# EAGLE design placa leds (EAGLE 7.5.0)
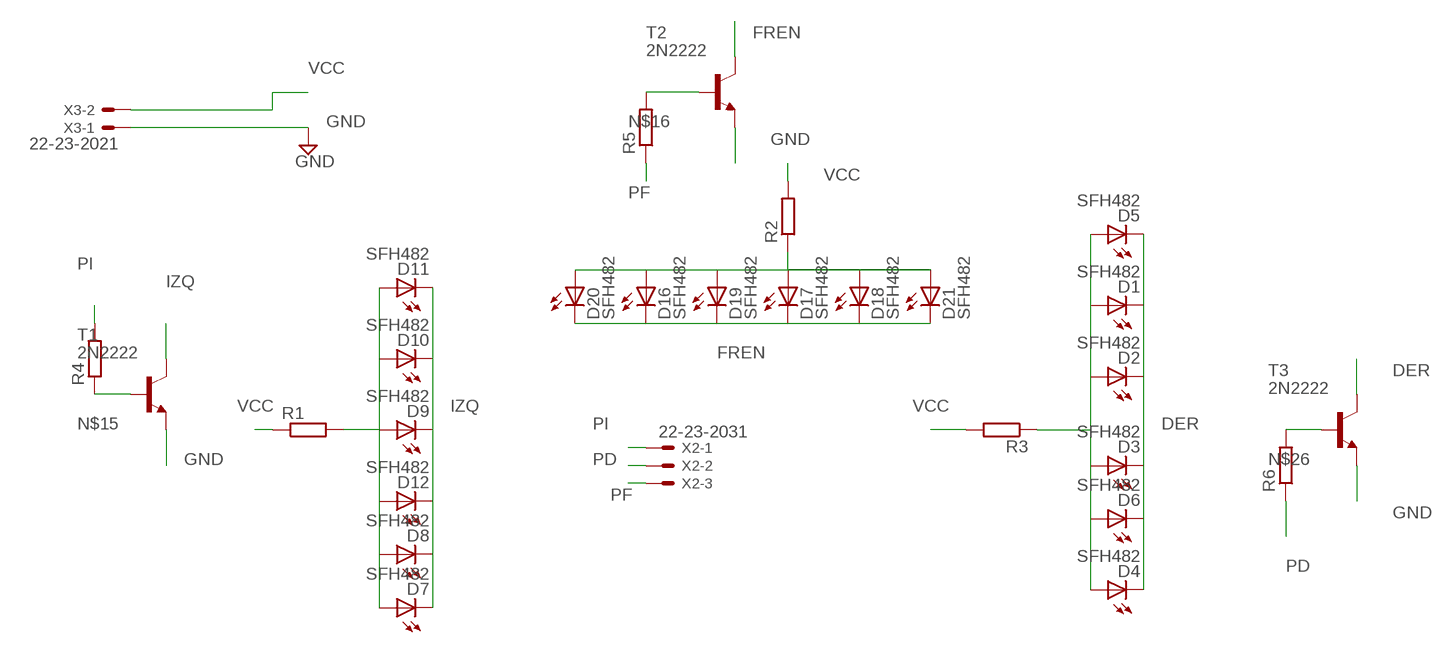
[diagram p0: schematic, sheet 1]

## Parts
D1  SFH482  [SFH482]
D2  SFH482  [SFH482]
D3  SFH482  [SFH482]
D4  SFH482  [SFH482]
D5  SFH482  [SFH482]
D6  SFH482  [SFH482]
D7  SFH482  [SFH482]
D8  SFH482  [SFH482]
D9  SFH482  [SFH482]
D10  SFH482  [SFH482]
D11  SFH482  [SFH482]
D12  SFH482  [SFH482]
D16  SFH482  [SFH482]
D17  SFH482  [SFH482]
D18  SFH482  [SFH482]
D19  SFH482  [SFH482]
D20  SFH482  [SFH482]
D21  SFH482  [SFH482]
R1  R-EU_VTA54  [VTA54]
R2  R-EU_VTA54  [VTA54]
R3  R-EU_VTA54  [VTA54]
R4  R-EU_0204/7  [0204/7]
R5  R-EU_0204/7  [0204/7]
R6  R-EU_0204/7  [0204/7]
T1  2N2222  [TO18]
T2  2N2222  [TO18]
T3  2N2222  [TO18]
X2  22-23-2031  [22-23-2031]
X3  22-23-2021  [22-23-2021]

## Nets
DER: D1.K(C) D2.K(C) D3.K(C) D4.K(C) D5.K(C) D6.K(C) T3.3(C)
FREN: D16.K(C) D17.K(C) D18.K(C) D19.K(C) D20.K(C) D21.K(C) T2.3(C)
GND: T1.1(E) T2.1(E) T3.1(E) X3.1
IZQ: D7.K(C) D8.K(C) D9.K(C) D10.K(C) D11.K(C) D12.K(C) T1.3(C)
N$2: D7.A D8.A D9.A D10.A D11.A D12.A R1.2
N$3: D16.A D17.A D18.A D19.A D20.A D21.A R2.1
N$4: D1.A D2.A D3.A D4.A D5.A D6.A R3.1
N$15: R4.1 T1.2(B)
N$16: R5.2 T2.2(B)
N$26: R6.2 T3.2(B)
PD: R6.1 X2.2
PF: R5.1 X2.3
PI: R4.2 X2.1
VCC: R1.1 R2.2 R3.2 X3.2

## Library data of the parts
D1-D12 D16-D21 = led:SFH482: IR LED
R1-R6 = resistor:R-EU_: RESISTOR, European symbol
T1-T3 = transistor:2N2222: NPN TRANSISTOR
X2 = con-molex:22-23-2031: .100" (2.54mm) Center Header - 3 Pin; MF: MOLEX; MPN: 22-23-2031; OC_FARNELL: 1462950; OC_NEWARK: 30C0862
X3 = con-molex:22-23-2021: .100" (2.54mm) Center Header - 2 Pin; MF: MOLEX; MPN: 22-23-2021; OC_FARNELL: 1462926; OC_NEWARK: 25C3832

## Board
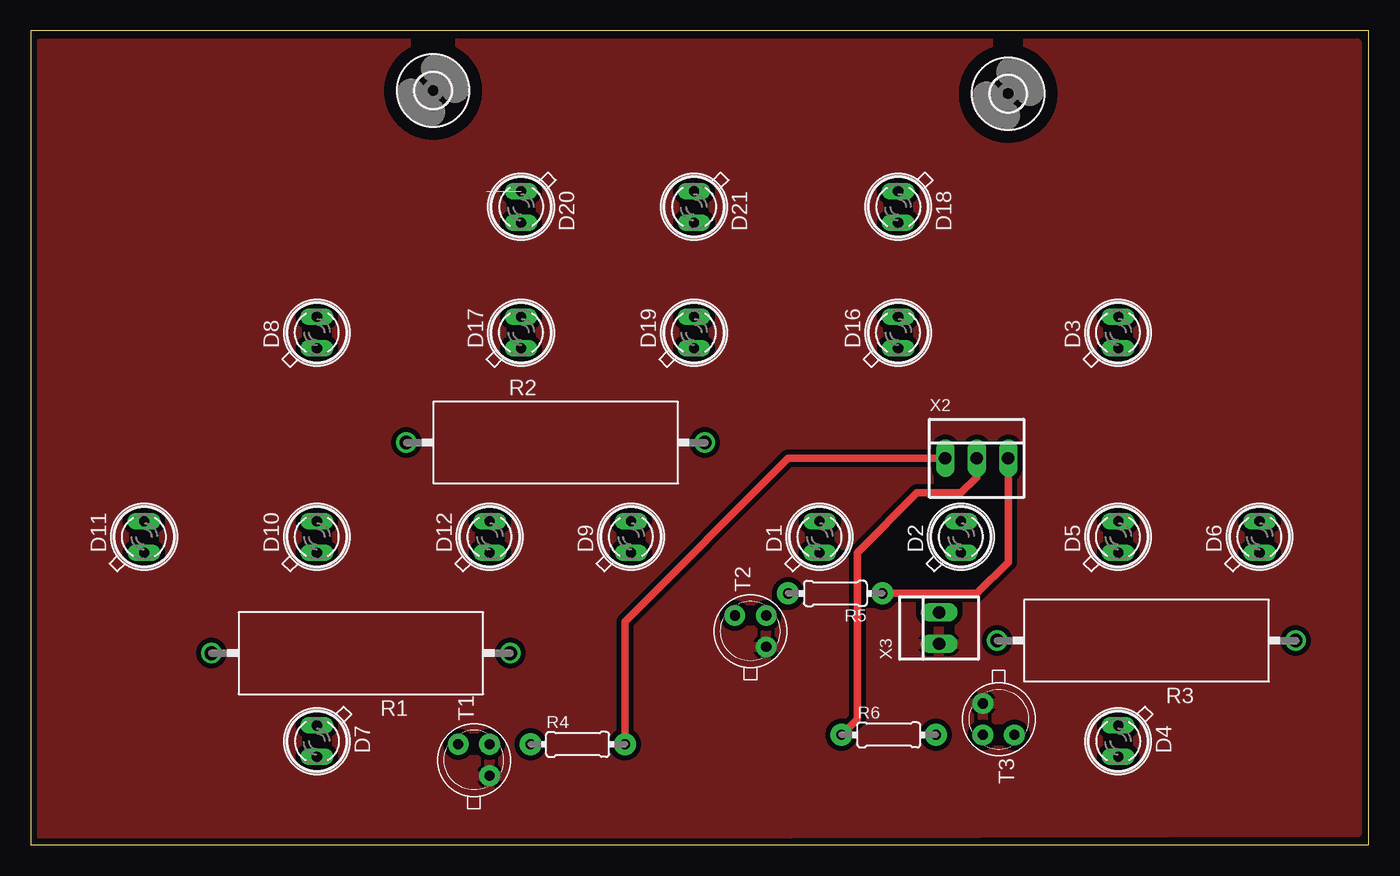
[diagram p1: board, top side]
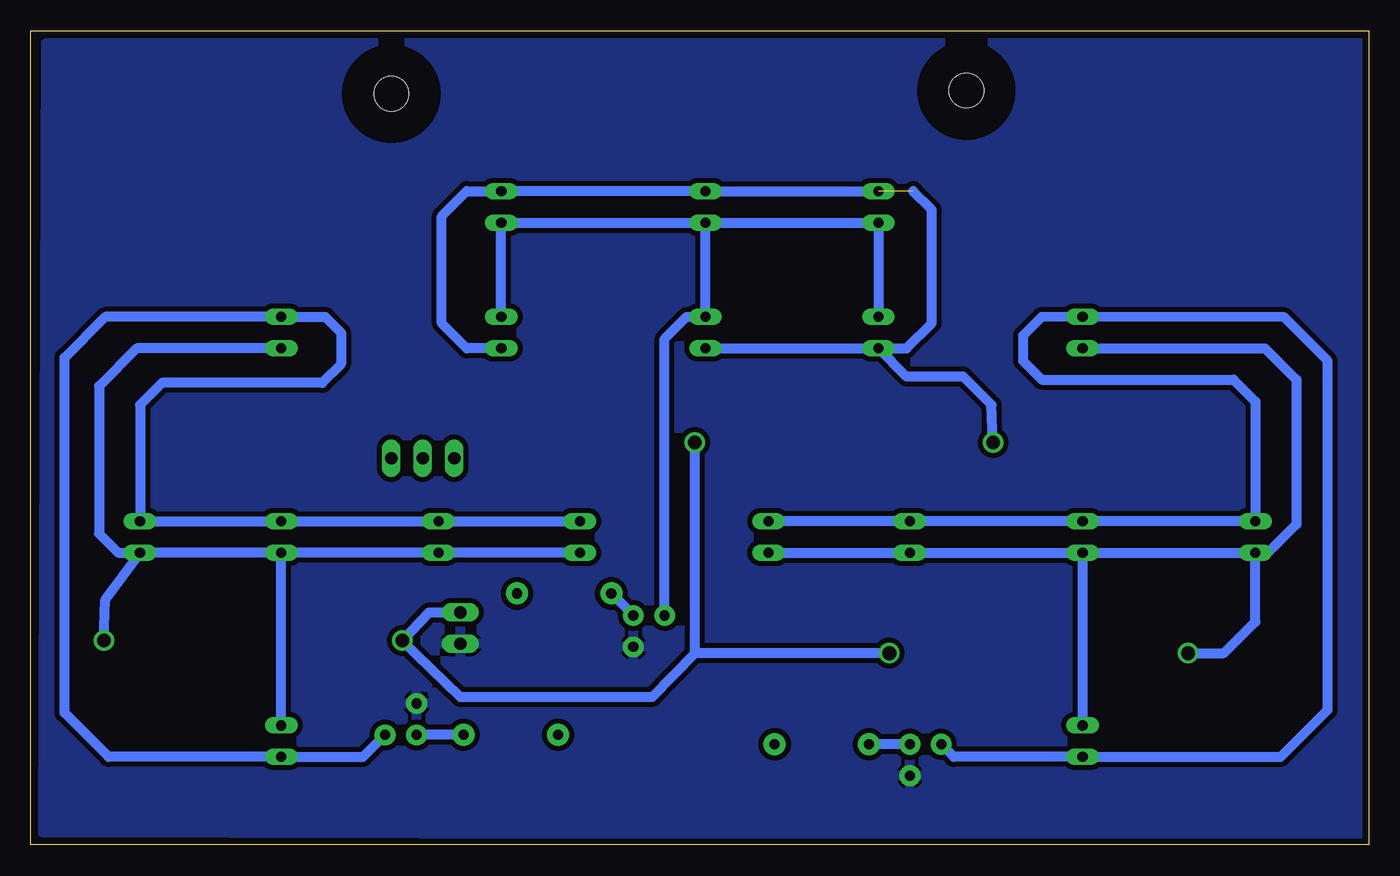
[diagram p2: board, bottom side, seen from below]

Size 108.13 x 65.78 mm. Coordinates in mm from the lower left corner, seen from the top.
Outline: 0,0 108.13,0 108.13,65.78 0,65.78 0,0
Copper layers (1*16): Top 0.035mm / dielectric 1.5mm / Bottom 0.035mm
Design rules "TE": minimum track width 12mil, minimum drill 23mil, track to track 10mil, track to pad 10mil, pad to pad 10mil, via to via 10mil, smd to smd 10mil, copper to edge 20mil, drill to drill 8mil, minimum pad ring 10mil, minimum via ring 8mil, stop-mask expansion 4mil, vias tented up to drill 0mil, thermal gap 10mil

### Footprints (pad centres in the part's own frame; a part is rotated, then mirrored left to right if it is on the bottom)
SFH482 = drill 0.813 long: A -1.27,0; K 1.27,0
VTA54 = drill 1.1: 1 -12.065,0; 2 12.065,0
0204/7 = drill 0.813 pad 1.778: 1 -3.81,0; 2 3.81,0
TO18 = drill 0.813 pad 1.676: 1 -1.27,-1.27; 2 1.27,-1.27; 3 1.27,1.27
2,8 = hole 2.8: 0,0
22-23-2031 = drill 1 long: 1 -2.54,0; 2 0,0; 3 2.54,0
22-23-2021 = drill 1 long: 1 -1.27,0; 2 1.27,0

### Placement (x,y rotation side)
D1  63.75,24.89 90 top
D2  75.18,24.89 90 top
D3  87.88,41.4 90 top
D4  87.88,8.38 270 top
D5  87.88,24.89 90 top
D6  99.31,24.89 90 top
D7  23.11,8.38 270 top
D8  23.11,41.4 90 top
D9  48.51,24.89 90 top
D10  23.11,24.89 90 top
D11  9.14,24.89 90 top
D12  37.08,24.89 90 top
D16  70.1,41.4 90 top
D17  39.62,41.4 90 top
D18  70.1,51.56 270 top
D19  53.59,41.4 90 top
D20  39.62,51.56 270 top
D21  53.59,51.56 270 top
R1  26.67,15.49 180 top
R2  42.42,32.51 0 top
R3  90.17,16.51 180 top
R4  44.2,8.13 0 top
R5  65.02,20.32 180 top
R6  69.34,8.89 0 top
T1  35.81,6.86 90 top
T2  58.17,17.27 90 top
T3  78.23,10.16 270 top
U$1  [2,8]  32.51,60.96 0 top
U$2  [2,8]  78.99,60.71 0 top
X2  76.45,31.24 0 top
X3  73.41,17.53 90 top

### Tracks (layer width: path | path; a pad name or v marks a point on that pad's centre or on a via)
DER
  Bottom 0.813: D1.K D2.K D5.K D6.K 99.31,35.56 97.54,37.34 84.58,37.34 83.06,38.86 83.06,41.4 84.33,42.67 D3.K 102.11,42.67 105.41,39.37 105.41,10.67 101.85,7.11 D4.K 81.28,7.11 T3.3
FREN
  Bottom 0.813: D16.K D18.K D21.K | D21.K D20.K D17.K | D21.K D19.K 55.12,42.67 56.9,40.89 T2.3
GND
  pour Bottom (isolate 0.406): 0.51,64.77 106.93,64.77 107.19,1.02 0.76,0.76
  pour Top (isolate 0.406): 0.76,64.77 107.19,64.77 107.19,1.02 0.76,0.76
IZQ
  Bottom 0.813: D9.K D12.K D10.K D11.K 9.14,35.81 10.92,37.59 26.42,37.59 27.94,39.12 27.94,41.15 26.42,42.67 23.64,42.64 | D8.K 23.64,42.64 | 23.64,42.64 6.86,42.67 3.3,39.12 3.3,10.92 7.11,7.11 D7.K 33.53,7.11 T1.3
N$2
  Bottom 0.813: D9.A D12.A D10.A | D10.A D11.A | D7.A D10.A | D8.A 8.38,40.13 5.84,37.59 5.84,25.91 8.13,23.62 D11.A | R1.2 11.68,15.49 9.14,18.03 D11.A
N$3  (1 unrouted)
  Bottom 0.813: D19.A D17.A | D17.A 37.34,40.13 35.31,42.16 35.31,51.31 36.83,52.83 | D20.A D21.A D18.A 72.9,52.83 74.93,50.8 74.93,42.16 72.9,40.13 D16.A | R2.1 30.48,35.56 32.77,37.85 37.34,37.85 D17.A
N$4
  Bottom 0.813: D1.A D2.A D5.A | D5.A D6.A | D3.A 99.57,40.13 102.62,37.08 102.62,25.15 101.09,23.62 D6.A | D4.A D5.A | R3.1 102.11,19.81 D6.A
N$15
  Bottom 0.813: T1.2 R4.1
N$16
  Bottom 0.813: T2.2 R5.2
N$26
  Bottom 0.813: R6.2 T3.2
PD
  Top 0.61: X2.2 76.45,29.72 75.18,28.45 71.63,28.45 66.8,23.62 66.8,10.16 R6.1
PF
  Top 0.61: X2.3 78.99,22.86 76.45,20.32 R5.1
PI
  Top 0.61: X2.1 61.21,31.24 48.01,18.03 R4.2
VCC
  Bottom 0.813: X3.2 75.95,18.8 R3.2 73.41,11.94 57.91,11.94 54.49,15.47 | R1.1 54.36,15.49 54.49,15.47 | R2.2 54.49,15.47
